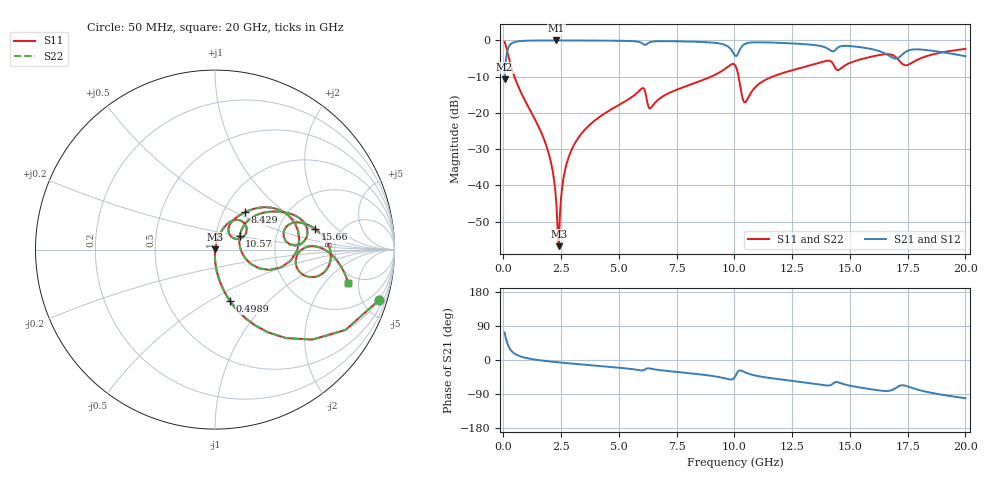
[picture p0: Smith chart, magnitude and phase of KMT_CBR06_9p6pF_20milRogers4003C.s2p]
! Data measured by Modelithics Inc. support@modelithics.com 813-866-6335
! KEMET CBR0603 9.6pF, Pad Width= 0.851mm, Pad Length= 0.64mm, Pad Gap= 0.62mm, 20mil Rogers 4003C substrate Data, January 2022
# hz S ma R 50
! 2 Port Network Data from SP1.SP block
! freq  magS11  angS11  magS21  angS21  magS12  angS12  magS22  angS22
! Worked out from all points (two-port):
!   401 points, 50 MHz to 20 GHz, reference 50 ohm
!   highest |S21| = -0.01 dB at 2.294 GHz (marker M1); lowest = -10.7 dB at 50 MHz (marker M2)
!   |S21| within 3 dB of the highest: 166.9 MHz to 9.906 GHz (9.74 GHz wide, 193 % of centre); 10.2 GHz to 14.25 GHz (4.054 GHz wide, 33.2 % of centre)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
!   lowest |S11| = -56.8 dB at 2.394 GHz (marker M3), VSWR 1.00, Z = 50.1 + j0.0604 ohm
!   |S11| at or under -10 dB: 474.3 MHz to 8.989 GHz (8.515 GHz wide, 180 % of centre); 10.18 GHz to 11.65 GHz (1.467 GHz wide, 13.4 % of centre)
!   |S22| runs from -56.8 to -0.4 dB; largest |S21 - S12| = 0
!   S11 on the Smith chart (normalised r, x): 50 MHz: 0.99, -6.53; 498.9 MHz: 0.99, -0.63; 8.429 GHz: 1.26, +0.57; 10.57 GHz: 1.30, +0.20; 15.66 GHz: 3.22, +1.10; 20 GHz: 4.13, -3.67
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5e7  0.9566 -17.0  0.291 72.9  0.291 72.9  0.9566 -17.0
2.99375e8  0.4754 -62.3  0.8791 27.6  0.8791 27.6  0.4754 -62.3
4.98875e8  0.3007 -73.7  0.953 16.2  0.953 16.2  0.3007 -73.7
1.895375e9  0.03226 -91.1  0.9983 -3.1  0.9983 -3.1  0.03226 -91.1
2.14475e9  0.0148 -90.1  0.9986 -4.7  0.9986 -4.7  0.0148 -90.1
2.294375e9  0.005403 -82.6  0.9987 -5.7  0.9987 -5.7  0.005403 -82.6
2.394125e9  0.001446 24.6  0.9987 -6.3  0.9987 -6.3  0.001446 24.6
2.74325e9  0.02025 78.0  0.9984 -8.3  0.9984 -8.3  0.02025 78.0
3.391625e9  0.05239 76.6  0.997 -11.8  0.997 -11.8  0.05239 76.6
5.985125e9  0.2167 47.9  0.9233 -27.6  0.9233 -27.6  0.2167 47.9
6.33425e9  0.115 40.6  0.942 -22.3  0.942 -22.3  0.115 40.6
6.73325e9  0.1552 59.2  0.9755 -26.3  0.9755 -26.3  0.1552 59.2
8.429e9  0.2686 51.1  0.9557 -37.3  0.9557 -37.3  0.2686 51.1
9.626e9  0.412 33.3  0.8568 -48.9  0.8568 -48.9  0.412 33.3
1.0025e10  0.4578 -0.7  0.6168 -44.3  0.6168 -44.3  0.4578 -0.7
1.037412e10  0.1508 -6.6  0.8596 -30.2  0.8596 -30.2  0.1508 -6.6
1.057362e10  0.1575 29.0  0.9216 -35.4  0.9216 -35.4  0.1575 29.0
1.336662e10  0.46 26.0  0.8693 -61.7  0.8693 -61.7  0.46 26.0
1.566088e10  0.5686 11.8  0.7884 -74.8  0.7884 -74.8  0.5686 11.8
1.670825e10  0.6441 -6.6  0.6122 -81.3  0.6122 -81.3  0.6441 -6.6
1.74065e10  0.4537 -7.7  0.6927 -67.8  0.6927 -67.8  0.4537 -7.7
2e10  0.7645 -14.0  0.6054 -101.0  0.6054 -101.0  0.7645 -14.0
